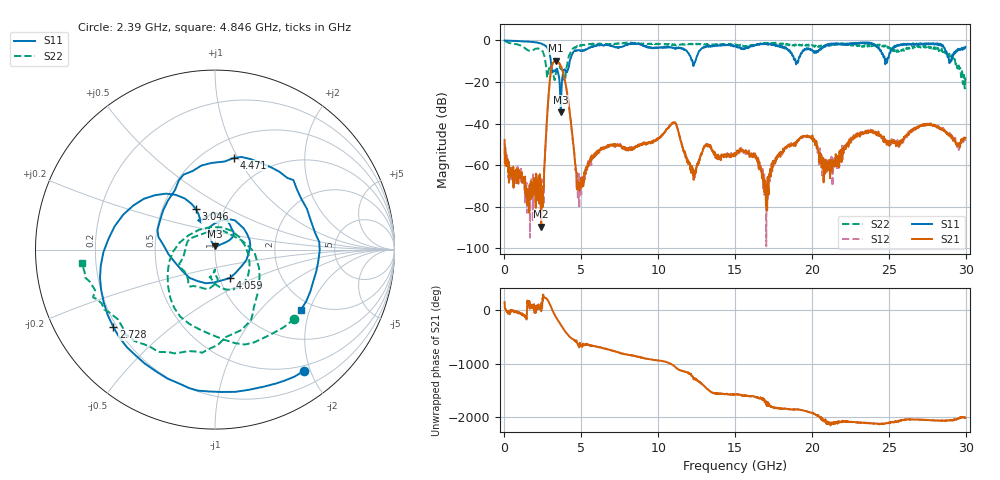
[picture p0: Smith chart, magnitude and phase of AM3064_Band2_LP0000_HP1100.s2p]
# Hz S DB R 50.0
!freq dBS11 angS11 dBS21 angS21 dBS12 angS12 dBS22 angS22
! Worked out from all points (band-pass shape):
!   1600 points, 10 MHz to 29.98 GHz, reference 50 ohm
!   highest |S21| = -9.80 dB at 3.328 GHz (marker M1); lowest = -89.5 dB at 2.39 GHz (marker M2)
!   |S21| within 3 dB of the highest: 3.069 GHz to 3.695 GHz (626.7 MHz wide, 18.5 % of centre)
!   lowest |S11| = -34.5 dB at 3.665 GHz (marker M3), VSWR 1.04, Z = 49.9 + j1.87 ohm
!   |S11| at or under -10 dB: 3.015 GHz to 4.243 GHz (1.227 GHz wide, 33.8 % of centre); 12.23 GHz to 12.41 GHz (180.7 MHz wide, 1.47 % of centre); 18.93 GHz to 19.11 GHz (178 MHz wide, 0.936 % of centre)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
!   |S22| runs from -23.1 to -0.2 dB; largest |S21 - S12| = 0.012
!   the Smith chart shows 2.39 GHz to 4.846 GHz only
!   S11 on the Smith chart (normalised r, x): 2.39 GHz: 0.42, -1.90; 2.728 GHz: 0.19, -0.33; 3.046 GHz: 0.74, +0.35; 4.059 GHz: 1.12, -0.37; 4.471 GHz: 0.69, +0.97; 4.846 GHz: 1.72, -1.75
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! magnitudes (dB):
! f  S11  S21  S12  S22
! 10 MHz  0.0  -47.9  -51.8  -0.2
! 2.39 GHz  -1.5  -89.5  -72.9  -4.6
! 2.728 GHz  -3.0  -42.6  -42.6  -13.9
! 3.046 GHz  -12.1  -13.6  -13.6  -14.7
! 3.328 GHz  -14.4  -9.8  -9.9  -16.4
! 3.665 GHz  -34.5  -12.4  -12.2  -13.3
! 4.059 GHz  -14.9  -24.5  -24.5  -12.3
! 4.471 GHz  -5.6  -49.6  -49.7  -3.8
! 4.846 GHz  -4.7  -69.7  -64.1  -2.6
! 5.015 GHz  -5.2  -66.0  -67.1  -2.5
! 6.289 GHz  -2.1  -52.0  -51.5  -1.7
! 10 GHz  -3.4  -47.2  -47.4  -1.7
! 11.09 GHz  -4.0  -39.6  -39.5  -1.9
! 12.29 GHz  -12.3  -62.9  -63.3  -1.5
! 13.15 GHz  -3.0  -50.1  -49.6  -2.1
! 15 GHz  -2.6  -55.5  -54.3  -1.9
! 17.03 GHz  -1.7  -69.7  -98.9  -1.3
! 17.78 GHz  -2.9  -55.2  -54.9  -1.5
! 19.99 GHz  -4.5  -47.2  -46.7  -2.2
! 20.91 GHz  -2.2  -61.0  -63.1  -2.4
! 25 GHz  -8.1  -50.5  -48.2  -3.1
! 29.98 GHz  -3.2  -46.9  -46.7  -17.3
